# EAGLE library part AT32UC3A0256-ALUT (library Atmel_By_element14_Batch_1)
32-Bit Microcontroller
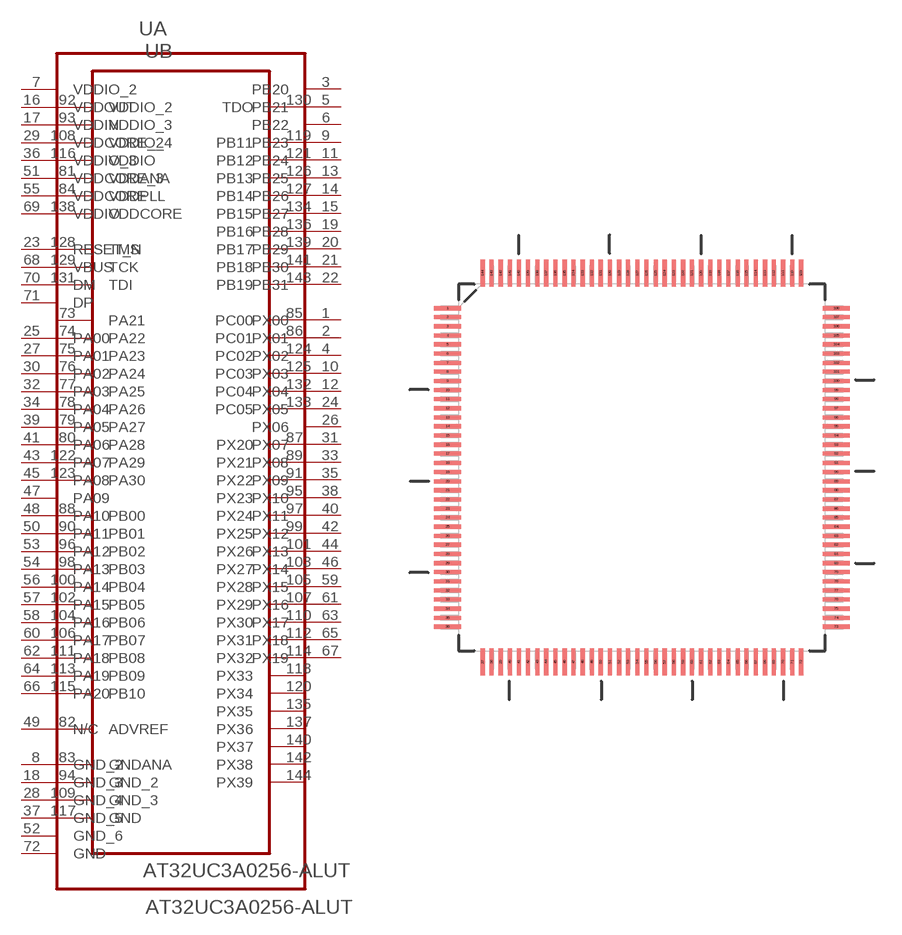
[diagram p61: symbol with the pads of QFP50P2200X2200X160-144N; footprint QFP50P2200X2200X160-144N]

Designator prefix U; gates A=AT32UC3A0256-ALUT_A B=AT32UC3A0256-ALUT_B

## AT32UC3A0256-ALUT (DESCRIPTION: 32-Bit Microcontroller; MPN: AT32UC3A0256-ALUT; OC_FARNELL: 1841635; OC_NEWARK: 12T1369; PACKAGE: LQFP-144; SUPPLIER: Atmel Corporation)  [QFP50P2200X2200X160-144N]
1  A:PX00
2  A:PX01
3  A:PB20
4  A:PX02
5  A:PB21
6  A:PB22
7  A:VDDIO_2  pwr
8  A:GND_2  pas
9  A:PB23
10  A:PX03
11  A:PB24
12  A:PX04
13  A:PB25
14  A:PB26
15  A:PB27
16  A:VDDOUT  pwr
17  A:VDDIN  pwr
18  A:GND_3  pas
19  A:PB28
20  A:PB29
21  A:PB30
22  A:PB31
23  A:RESET_N  in
24  A:PX05
25  A:PA00
26  A:PX06
27  A:PA01
28  A:GND_4  pas
29  A:VDDCORE_2  pwr
30  A:PA02
31  A:PX07
32  A:PA03
33  A:PX08
34  A:PA04
35  A:PX09
36  A:VDDIO_3  pwr
37  A:GND_5  pas
38  A:PX10
39  A:PA05
40  A:PX11
41  A:PA06
42  A:PX12
43  A:PA07
44  A:PX13
45  A:PA08
46  A:PX14
47  A:PA09
48  A:PA10
49  A:N/C  nc
50  A:PA11
51  A:VDDCORE_3  pwr
52  A:GND_6  pas
53  A:PA12
54  A:PA13
55  A:VDDCORE  pwr
56  A:PA14
57  A:PA15
58  A:PA16
59  A:PX15
60  A:PA17
61  A:PX16
62  A:PA18
63  A:PX17
64  A:PA19
65  A:PX18
66  A:PA20
67  A:PX19
68  A:VBUS  in
69  A:VDDIO  pwr
70  A:DM  in
71  A:DP  in
72  A:GND  pas
73  B:PA21
74  B:PA22
75  B:PA23
76  B:PA24
77  B:PA25
78  B:PA26
79  B:PA27
80  B:PA28
81  B:VDDANA  pwr
82  B:ADVREF  pas
83  B:GNDANA  pas
84  B:VDDPLL  pwr
85  B:PC00
86  B:PC01
87  B:PX20
88  B:PB00
89  B:PX21
90  B:PB01
91  B:PX22
92  B:VDDIO_2  pwr
93  B:VDDIO_3  pwr
94  B:GND_2  pas
95  B:PX23
96  B:PB02
97  B:PX24
98  B:PB03
99  B:PX25
100  B:PB04
101  B:PX26
102  B:PB05
103  B:PX27
104  B:PB06
105  B:PX28
106  B:PB07
107  B:PX29
108  B:VDDIO_4  pwr
109  B:GND_3  pas
110  B:PX30
111  B:PB08
112  B:PX31
113  B:PB09
114  B:PX32
115  B:PB10
116  B:VDDIO  pwr
117  B:GND  pas
118  B:PX33
119  B:PB11
120  B:PX34
121  B:PB12
122  B:PA29
123  B:PA30
124  B:PC02
125  B:PC03
126  B:PB13
127  B:PB14
128  B:TMS  in
129  B:TCK  in
130  B:TDO  out
131  B:TDI  in
132  B:PC04
133  B:PC05
134  B:PB15
135  B:PX35
136  B:PB16
137  B:PX36
138  B:VDDCORE  pwr
139  B:PB17
140  B:PX37
141  B:PB18
142  B:PX38
143  B:PB19
144  B:PX39

## Footprint QFP50P2200X2200X160-144N (pad centres in mm)
smd 1.473 x 0.229: 1 -10.668,8.738; 2 -10.668,8.255; 3 -10.668,7.747; 4 -10.668,7.239; 5 -10.668,6.756; 6 -10.668,6.248; 7 -10.668,5.74; 8 -10.668,5.258; 9 -10.668,4.75; 10 -10.668,4.242; 11 -10.668,3.759; 12 -10.668,3.251; 13 -10.668,2.743; 14 -10.668,2.261; 15 -10.668,1.753; 16 -10.668,1.245; 17 -10.668,0.762; 18 -10.668,0.254; 19 -10.668,-0.254; 20 -10.668,-0.762; 21 -10.668,-1.245; 22 -10.668,-1.753; 23 -10.668,-2.261; 24 -10.668,-2.743; 25 -10.668,-3.251; 26 -10.668,-3.759; 27 -10.668,-4.242; 28 -10.668,-4.75; 29 -10.668,-5.258; 30 -10.668,-5.74; 31 -10.668,-6.248; 32 -10.668,-6.756; 33 -10.668,-7.239; 34 -10.668,-7.747; 35 -10.668,-8.255; 36 -10.668,-8.738; 73 10.668,-8.738; 74 10.668,-8.255; 75 10.668,-7.747; 76 10.668,-7.239; 77 10.668,-6.756; 78 10.668,-6.248; 79 10.668,-5.74; 80 10.668,-5.258; 81 10.668,-4.75; 82 10.668,-4.242; 83 10.668,-3.759; 84 10.668,-3.251; 85 10.668,-2.743; 86 10.668,-2.261; 87 10.668,-1.753; 88 10.668,-1.245; 89 10.668,-0.762; 90 10.668,-0.254; 91 10.668,0.254; 92 10.668,0.762; 93 10.668,1.245; 94 10.668,1.753; 95 10.668,2.261; 96 10.668,2.743; 97 10.668,3.251; 98 10.668,3.759; 99 10.668,4.242; 100 10.668,4.75; 101 10.668,5.258; 102 10.668,5.74; 103 10.668,6.248; 104 10.668,6.756; 105 10.668,7.239; 106 10.668,7.747; 107 10.668,8.255; 108 10.668,8.738
smd 0.229 x 1.473: 37 -8.738,-10.668; 38 -8.255,-10.668; 39 -7.747,-10.668; 40 -7.239,-10.668; 41 -6.756,-10.668; 42 -6.248,-10.668; 43 -5.74,-10.668; 44 -5.258,-10.668; 45 -4.75,-10.668; 46 -4.242,-10.668; 47 -3.759,-10.668; 48 -3.251,-10.668; 49 -2.743,-10.668; 50 -2.261,-10.668; 51 -1.753,-10.668; 52 -1.245,-10.668; 53 -0.762,-10.668; 54 -0.254,-10.668; 55 0.254,-10.668; 56 0.762,-10.668; 57 1.245,-10.668; 58 1.753,-10.668; 59 2.261,-10.668; 60 2.743,-10.668; 61 3.251,-10.668; 62 3.759,-10.668; 63 4.242,-10.668; 64 4.75,-10.668; 65 5.258,-10.668; 66 5.74,-10.668; 67 6.248,-10.668; 68 6.756,-10.668; 69 7.239,-10.668; 70 7.747,-10.668; 71 8.255,-10.668; 72 8.738,-10.668; 109 8.738,10.668; 110 8.255,10.668; 111 7.747,10.668; 112 7.239,10.668; 113 6.756,10.668; 114 6.248,10.668; 115 5.74,10.668; 116 5.258,10.668; 117 4.75,10.668; 118 4.242,10.668; 119 3.759,10.668; 120 3.251,10.668; 121 2.743,10.668; 122 2.261,10.668; 123 1.753,10.668; 124 1.245,10.668; 125 0.762,10.668; 126 0.254,10.668; 127 -0.254,10.668; 128 -0.762,10.668; 129 -1.245,10.668; 130 -1.753,10.668; 131 -2.261,10.668; 132 -2.743,10.668; 133 -3.251,10.668; 134 -3.759,10.668; 135 -4.242,10.668; 136 -4.75,10.668; 137 -5.258,10.668; 138 -5.74,10.668; 139 -6.248,10.668; 140 -6.756,10.668; 141 -7.239,10.668; 142 -7.747,10.668; 143 -8.255,10.668; 144 -8.738,10.668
